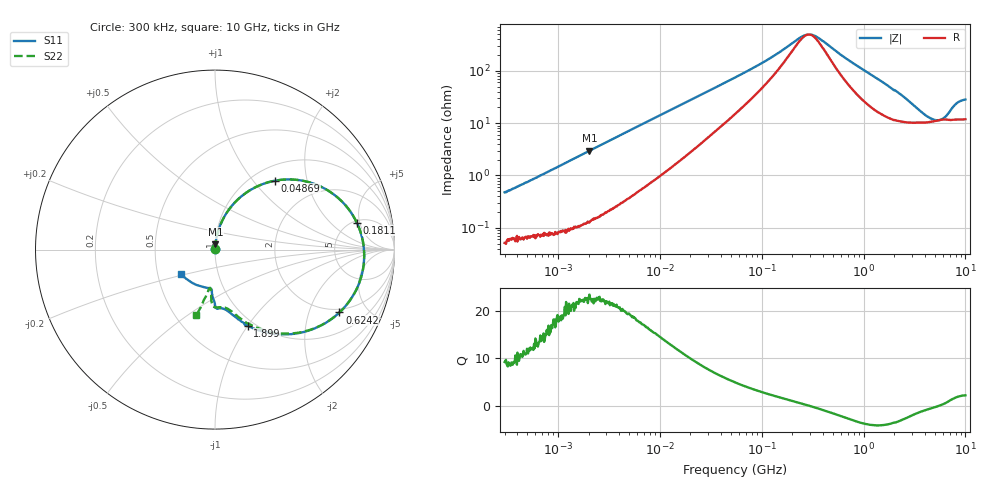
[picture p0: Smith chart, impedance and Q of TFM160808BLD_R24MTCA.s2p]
! S-Parameter Data Generated by TDK Corporation
! Copyright(C) 2024 TDK Corporation.
! All Rights Reserved.
! TDK P/N: TFM160808BLD-R24MTCA (SMD / SMT Inductor (Coil))
! Property: L=240nH at 1MHz
! Size(LxWxT): 1.6x0.8x0.8mm
! Model Type: s2p (Touchstone File Format Version 1.0)
! Frequency: DC=Yes Start=0.3MHz Stop=10000MHz 802points Log-sweep
! Model Generated on May 28, 2024
! Terms and conditions regarding TDK Simulation Models:
! 1)This simulation model is being provided solely for informational
!  purposes. Please refer to the specifications of the products in
!  terms of detailed characteristics of such products.
! 2)In no event shall TDK Corporation of any of its subsidiaries be
!  liable for any loss or damage arising, directly or indirectly,
!  from any information contained in this simulation model, including,
!  but not limited to loss or damages arising from any inaccuracies,
!  omissions or errors in connection with such information.
! 3)Any and all copyrights on this simulation model are owned by
!  TDK Corporation.  Duplication or redistribution of this simulation
!  model without prior written permission from TDK Corporation
!  is prohibited.
! 4)This simulation model is subject to any modification or change
!  without any prior notice.
! 5)Neither TDK Corporation nor any of its subsidiaries shall make any
!  warranty, express or implied, including but not limited to the
!  correctness, implied warranties of merchantability and fitness for
!  a particular purpose with respect to this simulation models.
! 6)The use of this simulation model shall be deemed to have consented
!  to the terms and conditions hereof.
! Port Assignments:
!  1 ---@@@--- 2
! Applicable Conditions:
!  Temperature = 25 degC
!  DC Bias Current = 0 A
!  Small Signal Operation
# Hz S MA R 50
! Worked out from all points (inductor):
!   801 points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, 300 kHz to 10 GHz, reference 50 ohm
!   read as one part in series: L = 242 nH near 318.3 kHz
!   highest Q = 22.5 at 2.04 MHz (marker M1), where L = 231 nH
!   self-resonance near 289.5 MHz
!   S11 on the Smith chart (normalised r, x): 300 kHz: 1.00, +0.01; 48.69 MHz: 1.25, +1.30; 181.1 MHz: 5.30, +4.51; 624.2 MHz: 1.83, -3.23; 1.899 GHz: 0.93, -1.00; 10 GHz: 0.66, -0.19
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300000  0.004915 84.3  0.9993 -0.3  0.9991 -0.2  0.005122 88.5
1713600  0.02489 86.0  0.9985 -1.4  0.9985 -1.4  0.02492 86.2
2040262  0.02946 85.7  0.9982 -1.7  0.9984 -1.7  0.02959 86.0
9671944  0.1333 78.4  0.9819 -7.7  0.9822 -7.7  0.1333 78.4
2.346945e7  0.2971 66.3  0.9223 -17.4  0.9225 -17.4  0.297 66.3
4.868606e7  0.5087 49.0  0.7724 -30.4  0.7726 -30.4  0.5087 49.0
5.477226e7  0.5452 45.7  0.7358 -32.7  0.736 -32.7  0.5451 45.7
9.444554e7  0.6955 29.6  0.5324 -42.1  0.5325 -42.1  0.6956 29.6
1.810762e8  0.8042 10.8  0.2744 -40.2  0.2744 -40.2  0.8043 10.8
2.569609e8  0.8288 0.9  0.1781 -16.8  0.1781 -16.8  0.829 1.0
3.126428e8  0.8325 -4.8  0.1706 7.6  0.1706 7.6  0.8328 -4.7
4.448526e8  0.8195 -15.4  0.2572 36.5  0.2572 36.5  0.8199 -15.3
6.242396e8  0.7768 -26.8  0.3974 40.9  0.3975 40.8  0.778 -26.5
1.054047e9  0.6515 -45.8  0.62 31.1  0.6201 31.1  0.6537 -45.1
1.767019e9  0.4861 -64.3  0.7774 15.3  0.7775 15.2  0.49 -62.1
1.898818e9  0.4627 -66.8  0.7929 12.8  0.793 12.8  0.4671 -64.2
2.720446e9  0.372 -75.3  0.8411 2.2  0.8413 2.1  0.3732 -73.1
3.682634e9  0.3304 -82.8  0.8527 -7.8  0.8529 -7.8  0.3265 -81.0
5.687864e9  0.3117 -89.9  0.845 -21.8  0.845 -21.8  0.3042 -93.0
7.875699e9  0.2239 -94.8  0.8549 -37.2  0.8547 -37.2  0.2146 -97.2
8.658336e9  0.2179 -101.4  0.8499 -43.1  0.8495 -43.2  0.2339 -99.4
1e10  0.2339 -144.5  0.7854 -54.4  0.7857 -54.5  0.3786 -105.9
